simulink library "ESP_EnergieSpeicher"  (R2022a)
settings: Solver=VariableStepAuto  StartTime=0.0  StopTime=10.0  RelTol=1e-3
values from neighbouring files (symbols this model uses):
  PAR_ESP_Anfangstemperatur = 10    [parameter_ESP.m]
  PAR_ESP_BTWirkungsgrad = 1.047    [parameter_ESP.m]
  PAR_ESP_Heizflaeche = 0.5    [parameter_ESP.m]
  PAR_ESP_ISO_Dicke = 0.08    [parameter_ESP.m]
  PAR_ESP_SMWirkungsgrad = 0.98    [parameter_ESP.m]
  PAR_ESP_VolumenWarmwasser = 50/1000    (= 0.05)    [parameter_ESP.m]
  PAR_ESP_Waermekap = 4200    [parameter_ESP.m]
  PAR_ESP_Wasserdichte = 1    [parameter_ESP.m]
  PAR_ESP_WLF_EPS = 0.032    [parameter_ESP.m]
libraries: $bdroot x1

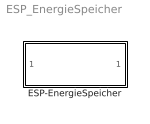
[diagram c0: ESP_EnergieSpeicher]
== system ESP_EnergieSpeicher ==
  ESP-EnergieSpeicher : Subsystem

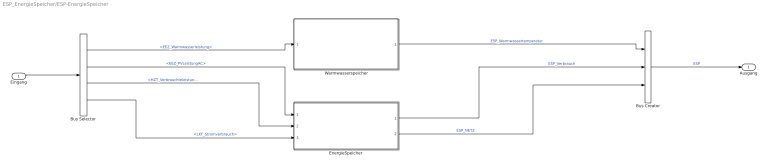
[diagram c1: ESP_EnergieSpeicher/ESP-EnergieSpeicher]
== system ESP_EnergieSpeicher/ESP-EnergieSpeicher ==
  Eingang : Inport
  Bus Creator : BusCreator  Inputs=3
  Bus Selector : BusSelector  OutputSignals=EEZ.EEZ_Warmwasserleistung,EEZ.EEZ_PVLeistungAC,HZT.HZT_Verbrauchteleistung,LKT.LKT_Stromverbrauch
  "EnergieSpeicher " : Subsystem
  Warmwasserspeicher : Subsystem
  Ausgang : Outport
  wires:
  Bus Creator/1 -> Ausgang/1  "ESP"
  Eingang/1 -> Bus Selector/1
  Bus Selector/1 -> Warmwasserspeicher/1(HZR_Heizleistung)  "<EEZ_Warmwasserleistung>"
  Warmwasserspeicher/1(ESP_Warmwassertemperatur) -> Bus Creator/1  "ESP_Warmwassertemperatur"
  "EnergieSpeicher "/1(ESP_Verbrauch) -> Bus Creator/2  "ESP_Verbrauch"
  "EnergieSpeicher "/2(ESP_NETZ) -> Bus Creator/3  "ESP_NETZ"
  Bus Selector/2 -> "EnergieSpeicher "/1(EEZ_PVLeistungAC)  "<EEZ_PVLeistungAC>"
  Bus Selector/3 -> "EnergieSpeicher "/2(LKT_LeistunglVerbrauch)  "<HZT_Verbrauchteleistung>"
  Bus Selector/4 -> "EnergieSpeicher "/3(HZT_LeistunglVerbrauch)  "<LKT_Stromverbrauch>"

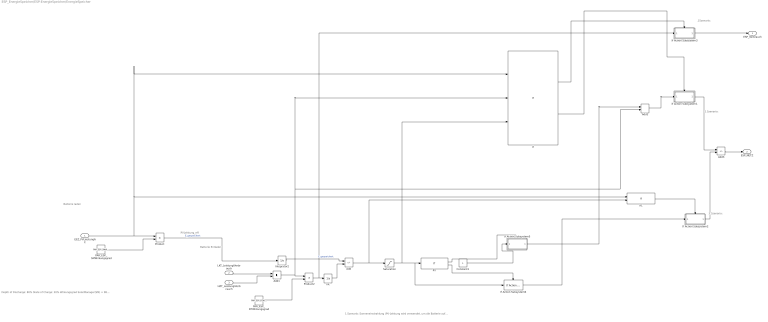
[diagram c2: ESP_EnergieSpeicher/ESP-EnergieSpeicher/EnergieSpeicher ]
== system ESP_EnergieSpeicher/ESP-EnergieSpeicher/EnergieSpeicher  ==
  note: 3.Szenario:
  note: 2.Szenario:
  note: .1Szenario:
  note: Batterie Iaden
  note: Depth of Discharge: 80% State of Charge: 20% Wirkungsgrad SolarManager(SM) = 98% Wirkungsgrad Batterie(BT): 95,3% Quelle: https://www.rct-power.com/de/newsreader-1393/batteriespeicher-lithium-eisenphosphat.html#:~:text=Der%20Wirkungsgrad%20einer%20LiFePO4%2DBatterie,zwischen%2093%20bis%2098%20Prozent. MPPT Laderegler kurz erklärt – Solar Swiss GmbH So laden Sie LiFePO4-Akkus auf？ – Creabest-De Practical aspects of electrophoretic deposition to produce commercially viable supercapacitor energy storage electrodes - RSC Advances (RSC Publishing) DOI:10.1039/D0RA09197A
  note: 1.Szenario: Sonneneinstrahlung (PV-Leistung wird verwendet, um die Batterie aufzuladen und den Verbrauch zu versorgen 2.Szenario: keine Sonneneinstrahlung (keine PV-Leistung verfügbar und Batterie leer, dann wird der Strom aus dem Netz bezogen ) 3.Szenario: Batterie vollständig aufgeladen und Sonneneinstrahlung ( überschüssige Strom ins Netz eingespeist)
  note: PVLeistung_eff
  note: Batterie Entladen
  EEZ_PVLeistungAC : Inport
  LKT_LeistunglVerbrauch : Inport  Port=2
  HZT_LeistunglVerbrauch : Inport  Port=3
  Add : Sum  Inputs=+-
  Add1 : Sum
  Add2 : Sum
  Add3 : Sum  Inputs=-+
  Constant1 : Constant
  If : If  NumInputs=3  IfExpression=u1 > u2 & u3 <=20160000  ElseIfExpressions=u1 < u2 & u3==5040000  ShowElse=off
  If Action Subsystem1 : Subsystem  TreatAsAtomicUnit=on
  If Action Subsystem2 : Subsystem  TreatAsAtomicUnit=on
  If Action Subsystem3 : Subsystem  TreatAsAtomicUnit=on
  If Action Subsystem5 : Subsystem  TreatAsAtomicUnit=on
  If Action Subsystem6 : $bdroot/ESP-EnergieSpeicher/EnergieSpeicher /If Action Subsystem5  SystemSampleTime=-1  VariantActivationTime=update diagram  Latency=0  AutoFrameSizeCalculation=off
  If1 : If  NumInputs=2  IfExpression=u1 > u2  ShowElse=off
  If2 : If  IfExpression=u1 ==5040000
  Int. : Integrator
  Integrator2 : Integrator
  PAR_ESP_BTWirkungsgrad : Constant  Value=PAR_ESP_BTWirkungsgrad
  PAR_ESP_SMWirkungsgrad : Constant  Value=PAR_ESP_SMWirkungsgrad
  Product : Product
  Product2 : Product
  Saturation : Saturate  UpperLimit=20160000  LowerLimit=5040000
  ESP_Verbrauch : Outport
  ESP_NETZ : Outport  Port=2
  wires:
  EEZ_PVLeistungAC/1 -> If/1, If1/1, Product/1
  Product/1 -> Integrator2/1  "E_gespeichert"
  Add1/1 -> If/2, Add2/2, Product2/1
  Add/1 -> If1/2, Saturation/1
  PAR_ESP_BTWirkungsgrad/1 -> Product2/2
  Saturation/1 -> If/3, If Action Subsystem6/1, If2/1
  HZT_LeistunglVerbrauch/1 -> Add1/2
  LKT_LeistunglVerbrauch/1 -> Add1/1
  PAR_ESP_SMWirkungsgrad/1 -> Product/2
  Integrator2/1 -> Add/1  "E_gespeichert"
  Product2/1 -> If Action Subsystem3/1(In1), Int./1
  Int./1 -> Add/2
  If2/1 -> If Action Subsystem5/Action
  Constant1/1 -> If Action Subsystem5/1(In1)
  If2/2 -> If Action Subsystem6/Action
  If/2 -> If Action Subsystem1/Action
  If/1 -> If Action Subsystem3/Action
  Add2/1 -> If Action Subsystem1/1(In1)
  If1/1 -> If Action Subsystem2/Action
  If Action Subsystem5/1(Out1) -> Add2/1
  If Action Subsystem6/1 -> If Action Subsystem2/1(In1)
  If Action Subsystem3/1(Out1) -> ESP_Verbrauch/1
  Add3/1 -> ESP_NETZ/1
  If Action Subsystem1/1(Out1) -> Add3/1
  If Action Subsystem2/1(Out1) -> Add3/2

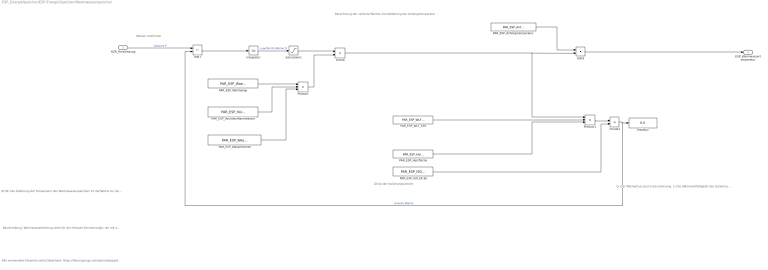
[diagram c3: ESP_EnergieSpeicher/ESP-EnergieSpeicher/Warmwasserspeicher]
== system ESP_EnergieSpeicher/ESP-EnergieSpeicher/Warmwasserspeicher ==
  note: Berechnung der verluste Wärme und Addierung der Anfangstemperatur
  note: Beschreibung: Warmwasserleistung steht für die erfasste Sonneenergie, die mit einen Schwellenwert (Soll_Leistung mit Gesamtwärmverlust) vergliechen werden, wenn z.B. im Sommer Sonne ausreichend sind, dann wird die Leistung durch den Integrator als zugeführte Wärme Q berechnet, mit der Formel wird die Temperaturdifferenz ausgegeben. Steht bei schlechterem Wetter nicht genügend Sonnenenergie zur Verfügung, diese Abweichung erfolgt über eine zweite Heizspirale im Speicher die Nacherwärmung des Wassers über das Heizgerät. Durch die Isolierung des Speichers wird der Wärmeverlust minimiert, sodass das Wasser über einen längeren Zeitraum warm gehalten werden kann.
  note: Wasser erwärmen
  note: dT/dt: Die Änderung der Temperatur des Warmwasserspeichers im Verhältnis zur Zeit. T: Die Temperatur des Warmwasserspeichers. m: Die Masse des Wassers im Warmwasserspeicher. c: Die spezifische Wärmekapazität des Wassers Q: Die Wärme, die dem Stoff zugeführt
  note: Q: Der Wärmefluss durch die Isolierung. λ: Die Wärmeleitfähigkeit des Isoliermaterials. A: Die Fläche der Isolierung. ΔT: Die Temperaturdifferenz zwischen dem Warmwasserspeicher und der Umgebung. d: Die Dicke der Isolierungsschicht.
  note: Alle verwendete Paramter sehe Datasheet: https://flamcogroup.com/de/catalog/pufferspeicher-und-warmwasserbereitung/warmwasserbereiter/standspeicher-flextherm-duo/flextherm-duo-120-500/18501/groups/g+c+p+a+nr+view Quelle für die Wärmleitfähigkeit der Expandiertes Polystyrol https://mit-sicherheit-eps.de/acht-gruende-fuer-eps
  note: Dicke der Isolierungsschicht
  HZR_Heizleistung : Inport
  Add1 : Sum  Inputs=+-
  Add3 : Sum
  Display2 : Display
  Divide : Product  Inputs=*/
  Divide1 : Product  Inputs=*/
  Integrator : Integrator
  PAR_ESP_Anfangstemperatur : Constant  Value=PAR_ESP_Anfangstemperatur
  PAR_ESP_Heizfläche : Constant  Value=PAR_ESP_Heizflaeche
  PAR_ESP_ISO_Dicke : Constant  Value=PAR_ESP_ISO_Dicke
  PAR_ESP_VolumenWarmwasser : Constant  Value=PAR_ESP_VolumenWarmwasser
  PAR_ESP_WLF_EPS : Constant  Value=PAR_ESP_WLF_EPS
  PAR_ESP_Wasserdichte : Constant  Value=PAR_ESP_Wasserdichte
  PAR_ESP_Wärmekap : Constant  Value=PAR_ESP_Waermekap
  Product : Product  Inputs=3
  Product1 : Product  Inputs=3
  Saturation1 : Saturate  UpperLimit=25000  LowerLimit=-1000
  ESP_Warmwassertemperatur : Outport
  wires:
  Add3/1 -> ESP_Warmwassertemperatur/1
  Integrator/1 -> Saturation1/1  "zugeführrte Wärme Q"
  PAR_ESP_ISO_Dicke/1 -> Divide1/2
  PAR_ESP_WLF_EPS/1 -> Product1/2
  Product/1 -> Divide/2
  Divide/1 -> Product1/1, Add3/2
  Saturation1/1 -> Divide/1
  PAR_ESP_Anfangstemperatur/1 -> Add3/1
  Product1/1 -> Divide1/1
  PAR_ESP_Wasserdichte/1 -> Product/3
  PAR_ESP_Wärmekap/1 -> Product/1
  Add1/1 -> Integrator/1
  PAR_ESP_VolumenWarmwasser/1 -> Product/2
  PAR_ESP_Heizfläche/1 -> Product1/3
  HZR_Heizleistung/1 -> Add1/1  "Leistung P"
  Divide1/1 -> Add1/2, Display2/1  "verluste Wärme"

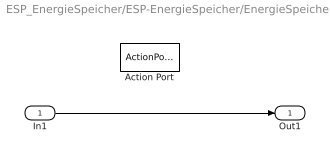
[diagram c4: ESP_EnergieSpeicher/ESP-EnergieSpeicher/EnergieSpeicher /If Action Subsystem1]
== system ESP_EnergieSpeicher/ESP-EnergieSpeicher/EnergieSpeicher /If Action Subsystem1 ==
  In1 : Inport
  Action Port : ActionPort
  Out1 : Outport
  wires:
  In1/1 -> Out1/1

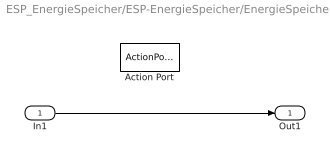
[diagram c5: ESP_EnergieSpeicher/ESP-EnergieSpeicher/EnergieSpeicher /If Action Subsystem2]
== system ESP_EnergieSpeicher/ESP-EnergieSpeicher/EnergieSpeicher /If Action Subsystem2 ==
  In1 : Inport
  Action Port : ActionPort
  Out1 : Outport
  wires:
  In1/1 -> Out1/1

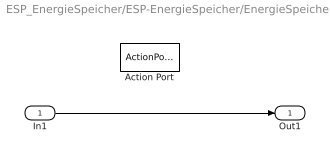
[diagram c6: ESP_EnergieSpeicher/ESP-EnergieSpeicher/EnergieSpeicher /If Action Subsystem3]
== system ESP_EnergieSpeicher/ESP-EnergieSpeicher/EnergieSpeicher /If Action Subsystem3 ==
  In1 : Inport
  Action Port : ActionPort
  Out1 : Outport
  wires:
  In1/1 -> Out1/1

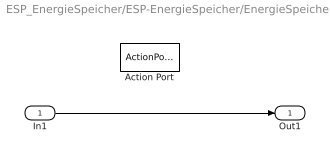
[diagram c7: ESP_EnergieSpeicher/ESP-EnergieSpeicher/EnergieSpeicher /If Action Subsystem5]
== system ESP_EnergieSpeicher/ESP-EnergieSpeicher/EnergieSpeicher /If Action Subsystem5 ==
  In1 : Inport
  Action Port : ActionPort
  Out1 : Outport
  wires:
  In1/1 -> Out1/1
